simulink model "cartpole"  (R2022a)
settings: Solver=FixedStepAuto  StartTime=0.0  StopTime=20  FixedStep=Tsim  RelTol=1e-3
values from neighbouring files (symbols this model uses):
  A = [0,1,0,0 ; 0,-d1, -g*m/M,0 ; 0,0,0,1 ; 0,d1/L,q_,-d2]    [cartpole_main.m]    (also in cp_kalman.m; time_varying_LQR.m = [0,1,0,0 ; 0,-d1,f_23, f_24; 0,0,0,1; 0, f_42, f_43, f_44 ]; cp_kalman_extended.m = [0,1,0,0 ; 0,-d1,f_23, f_24; 0,0,0,1; 0, f_42, f_43, f_44 ])
  B = [0, 1.0/M, 0., -1/(M*L)].'    [cartpole_main.m]    (also in cp_kalman.m; time_varying_LQR.m = [0; cp_kalman_extended.m = [0)
  C = [1,0,0,0;0,0,1,0]    [cartpole_main.m]
  P_k_init = .01    (= 0.01)    [cartpole_main.m]
  q1 = 5e-4    (= 0.0005)    [cartpole_main.m]    (also in loop_loader.m = const(3); rob_fc.m = const(3); loop_loader_ex.m = const(3))
  q2 = 1e-3    (= 0.001)    [cartpole_main.m]    (also in loop_loader.m = const(4); rob_fc.m = const(4); loop_loader_ex.m = const(4))
  Q_ctrl = diag([10,5,20,10])    [cartpole_main.m]
  r1 = 3e-4    (= 0.0003)    [cartpole_main.m]    (also in loop_loader.m = const(1); rob_fc.m = xx; loop_loader_ex.m = const(1))
  r2 = 2e-4    (= 0.0002)    [cartpole_main.m]    (also in loop_loader.m = const(2); rob_fc.m = const(2); loop_loader_ex.m = const(2))
  R_ctrl = 10    [cartpole_main.m]
  Ts = 0.01    [cartpole_main.m]    (also in loop_loader.m; cp_kalman.m = in(4); rob_fc.m; time_varying_LQR.m = in(11))
  x0 = [0,0,0.5, 0.1]    [cartpole_main.m]
undefined symbols (not defined in the file or in its folder): K_lqr
libraries: simulink x3

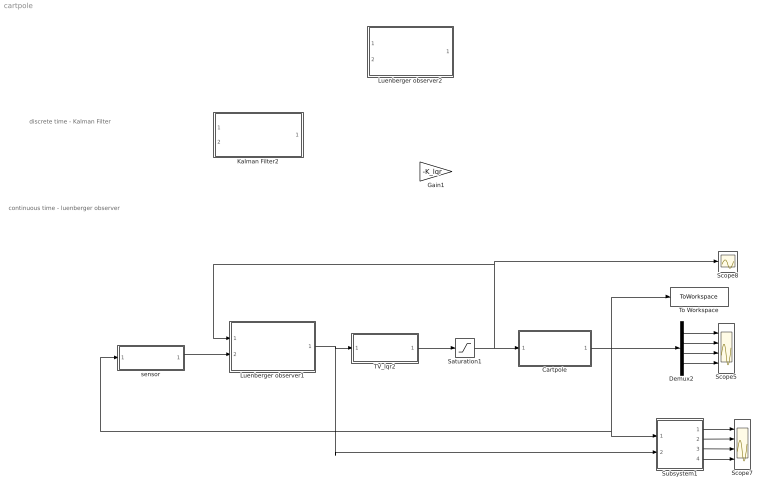
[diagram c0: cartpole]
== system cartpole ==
  note: continuous time - luenberger observer
  note: discrete time - Kalman Filter
  Cartpole : Subsystem
  Demux2 : Demux
  Gain1 : Gain  Commented=on  Gain=-K_lqr  Multiplication=Matrix(K*u)
  Kalman Filter2 : Subsystem  Commented=on  TreatAsAtomicUnit=on  SystemSampleTime=Ts
  Luenberger observer1 : Subsystem
  Luenberger observer2 : Subsystem  Commented=on
  Saturation1 : Saturate  UpperLimit=10  LowerLimit=-10
  Scope5 : Scope  NumInputPorts=4
  Scope7 : Scope  NumInputPorts=4
  Scope8 : Scope
  Subsystem1 : Subsystem
  TV_lqr2 : Subsystem  TreatAsAtomicUnit=on  SystemSampleTime=Ts
  To Workspace : ToWorkspace  VariableName=simout  SaveFormat=Timeseries  SampleTime=-1
  sensor : Subsystem
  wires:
  Subsystem1/1(x1) -> Scope7/1
  Subsystem1/3(x3) -> Scope7/3
  Subsystem1/4(x4) -> Scope7/4
  Subsystem1/2(x2) -> Scope7/2
  Demux2/4 -> Scope5/4
  Demux2/3 -> Scope5/3
  Demux2/2 -> Scope5/2
  Demux2/1 -> Scope5/1
  Saturation1/1 -> Scope8/1, Luenberger observer1/1(u), Cartpole/1(u)
  Luenberger observer1/1(x_hat) -> Subsystem1/2(x_hat), TV_lqr2/1(x)
  TV_lqr2/1(u) -> Saturation1/1
  Cartpole/1(x) -> Demux2/1, To Workspace/1, sensor/1(x), Subsystem1/1(x)
  sensor/1(y) -> Luenberger observer1/2(y)

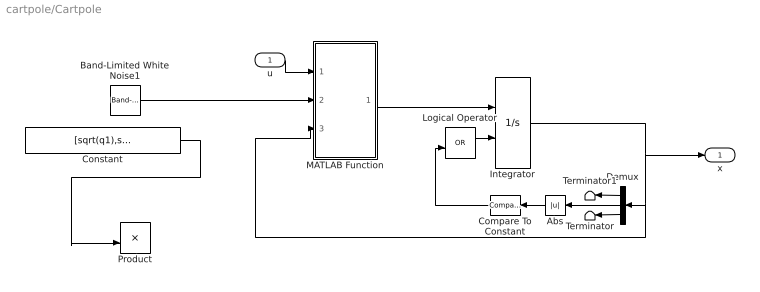
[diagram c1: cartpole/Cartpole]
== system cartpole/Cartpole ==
  u : Inport
  Abs : Abs  Commented=on
  Band-Limited White Noise1 : simulink/Sources/Band-Limited White Noise  Cov=[r1,r2]  Ts=Ts  seed=[23341]
  Compare To Constant : simulink/Logic and Bit Operations/Compare To Constant  Commented=on  relop=>=  const=1  OutDataTypeStr=boolean
  Constant : Constant  Commented=on  Value=[sqrt(q1),sqrt(q2)]
  Demux : Demux  Commented=on  Outputs=[2,1,1]
  Integrator : Integrator  ExternalReset=rising  InitialCondition=x0
  Logical Operator : Logic  Commented=on  Operator=OR  AllPortsSameDT=off  OutDataTypeStr=boolean
  MATLAB Function : MATLAB Function  TreatAsAtomicUnit=on
  Product : Product  Commented=on
  Terminator : Terminator
  Terminator1 : Terminator
  x : Outport
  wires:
  MATLAB Function/1(y) -> Integrator/1
  Integrator/1 -> x/1, MATLAB Function/3(s), Demux/1
  u/1 -> MATLAB Function/1(u)
  Compare To Constant/1 -> Logical Operator/2
  Demux/3 -> Terminator/1
  Demux/1 -> Terminator1/1
  Demux/2 -> Abs/1
  Abs/1 -> Compare To Constant/1
  Logical Operator/1 -> Integrator/2
  Constant/1 -> Product/2
  Band-Limited White Noise1/1 -> MATLAB Function/2(n)

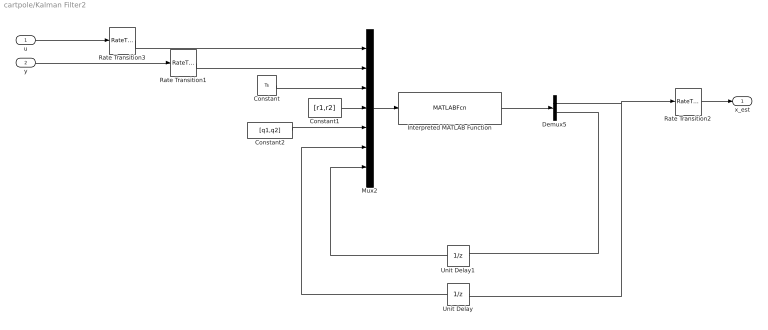
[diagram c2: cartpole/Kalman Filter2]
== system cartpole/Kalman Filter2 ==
  u : Inport
  y : Inport  Port=2
  Constant : Constant  Value=Ts
  Constant1 : Constant  Value=[r1,r2]
  Constant2 : Constant  Value=[q1,q2]
  Demux5 : Demux  Outputs=[4, 16]
  Interpreted MATLAB Function : MATLABFcn  MATLABFcn=cp_kalman  OutputDimensions=20
  Mux2 : Mux  Inputs=7
  Rate Transition1 : RateTransition  OutPortSampleTime=Ts
  Rate Transition2 : RateTransition
  Rate Transition3 : RateTransition  OutPortSampleTime=Ts
  Unit Delay : UnitDelay  InitialCondition=x0  SampleTime=-1  HasFrameUpgradeWarning=on
  Unit Delay1 : UnitDelay  InitialCondition=reshape( P_k_init*eye(4),[16,1])  SampleTime=-1  HasFrameUpgradeWarning=on
  x_est : Outport
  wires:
  Unit Delay1/1 -> Mux2/7
  Demux5/1 -> Rate Transition2/1, Unit Delay/1
  y/1 -> Rate Transition1/1
  Demux5/2 -> Unit Delay1/1
  Interpreted MATLAB Function/1 -> Demux5/1
  u/1 -> Rate Transition3/1
  Unit Delay/1 -> Mux2/6
  Mux2/1 -> Interpreted MATLAB Function/1
  Constant/1 -> Mux2/3
  Constant1/1 -> Mux2/4
  Constant2/1 -> Mux2/5
  Rate Transition3/1 -> Mux2/1
  Rate Transition1/1 -> Mux2/2
  Rate Transition2/1 -> x_est/1

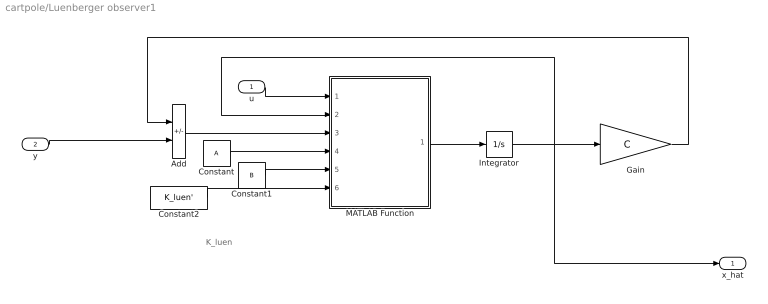
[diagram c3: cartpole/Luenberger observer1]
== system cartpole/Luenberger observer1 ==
  note: K_luen
  u : Inport
  y : Inport  Port=2
  Add : Sum  Inputs=-+
  Constant : Constant  Value=A
  Constant1 : Constant  Value=B
  Constant2 : Constant  Value=K_luen'
  Gain : Gain  Gain=C  Multiplication=Matrix(K*u)
  Integrator : Integrator  InitialCondition=[0,0,0,0]
  MATLAB Function : MATLAB Function  TreatAsAtomicUnit=on
  x_hat : Outport
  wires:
  y/1 -> Add/2
  u/1 -> MATLAB Function/1(u)
  Add/1 -> MATLAB Function/3(e)
  Gain/1 -> Add/1
  Integrator/1 -> x_hat/1, Gain/1, MATLAB Function/2(x)
  MATLAB Function/1(x_dot) -> Integrator/1
  Constant2/1 -> MATLAB Function/6(L)
  Constant1/1 -> MATLAB Function/5(B)
  Constant/1 -> MATLAB Function/4(A)

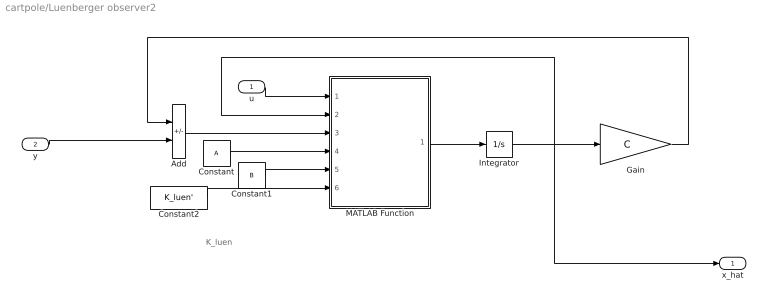
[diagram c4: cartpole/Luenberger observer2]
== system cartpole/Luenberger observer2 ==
  note: K_luen
  u : Inport
  y : Inport  Port=2
  Add : Sum  Inputs=-+
  Constant : Constant  Value=A
  Constant1 : Constant  Value=B
  Constant2 : Constant  Value=K_luen'
  Gain : Gain  Gain=C  Multiplication=Matrix(K*u)
  Integrator : Integrator  InitialCondition=[0,0,0,0]
  MATLAB Function : MATLAB Function  TreatAsAtomicUnit=on
  x_hat : Outport
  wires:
  y/1 -> Add/2
  u/1 -> MATLAB Function/1(u)
  Add/1 -> MATLAB Function/3(e)
  Gain/1 -> Add/1
  Integrator/1 -> x_hat/1, Gain/1, MATLAB Function/2(x)
  MATLAB Function/1(x_dot) -> Integrator/1
  Constant2/1 -> MATLAB Function/6(L)
  Constant1/1 -> MATLAB Function/5(B)
  Constant/1 -> MATLAB Function/4(A)

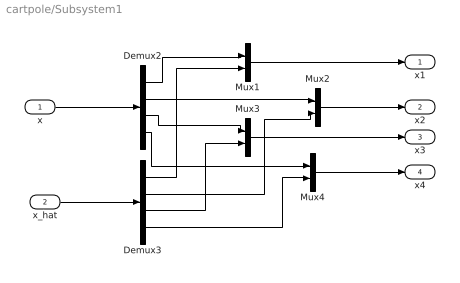
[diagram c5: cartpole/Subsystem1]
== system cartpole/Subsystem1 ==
  x : Inport
  x_hat : Inport  Port=2
  Demux2 : Demux
  Demux3 : Demux
  Mux{1..4} (4 alike) : Mux  Inputs=2
  x1 : Outport
  x2 : Outport  Port=2
  x3 : Outport  Port=3
  x4 : Outport  Port=4
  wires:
  Demux2/3 -> Mux3/1
  Demux3/4 -> Mux4/2
  x/1 -> Demux2/1
  Mux2/1 -> x2/1
  Demux2/1 -> Mux1/1
  x_hat/1 -> Demux3/1
  Demux3/2 -> Mux2/2
  Demux2/4 -> Mux4/1
  Demux3/3 -> Mux3/2
  Demux2/2 -> Mux2/1
  Mux3/1 -> x3/1
  Demux3/1 -> Mux1/2
  Mux4/1 -> x4/1
  Mux1/1 -> x1/1

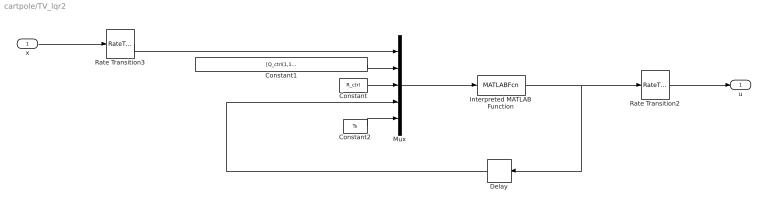
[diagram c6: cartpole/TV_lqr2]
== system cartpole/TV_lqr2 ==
  x : Inport
  Constant : Constant  Value=R_ctrl
  Constant1 : Constant  Value=[Q_ctrl(1,1),Q_ctrl(2,2),Q_ctrl(3,3),Q_ctrl(4,4)]
  Constant2 : Constant  Value=Ts
  Delay : Delay  DelayLength=1  InitialCondition=0
  Interpreted MATLAB Function : MATLABFcn  MATLABFcn=time_varying_LQR
  Mux : Mux  Inputs=5
  Rate Transition2 : RateTransition
  Rate Transition3 : RateTransition  OutPortSampleTime=Ts
  u : Outport
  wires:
  Constant2/1 -> Mux/5
  Rate Transition2/1 -> u/1
  Rate Transition3/1 -> Mux/1
  Delay/1 -> Mux/4
  Constant1/1 -> Mux/2
  Constant/1 -> Mux/3
  Mux/1 -> Interpreted MATLAB Function/1
  x/1 -> Rate Transition3/1
  Interpreted MATLAB Function/1 -> Rate Transition2/1, Delay/1

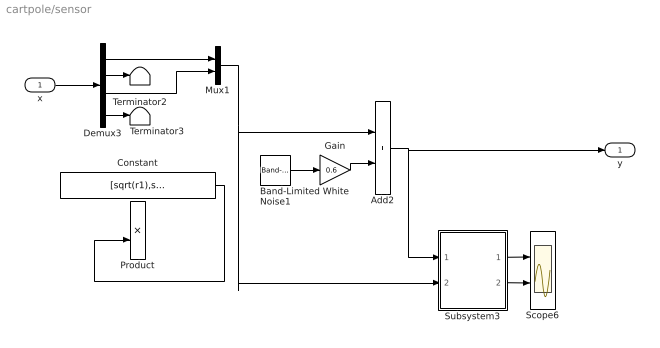
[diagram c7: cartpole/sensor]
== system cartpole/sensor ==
  x : Inport
  Add2 : Sum
  Band-Limited White Noise1 : simulink/Sources/Band-Limited White Noise  Cov=[r1,r2]  Ts=Ts  seed=[8451]
  Constant : Constant  Commented=on  Value=[sqrt(r1),sqrt(r2)]
  Demux3 : Demux
  Gain : Gain  Gain=0.6
  Mux1 : Mux  Inputs=2
  Product : Product  Commented=on
  Scope6 : Scope  NumInputPorts=2
  Subsystem3 : Subsystem
  Terminator2 : Terminator
  Terminator3 : Terminator
  y : Outport
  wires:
  Demux3/4 -> Terminator3/1
  Demux3/2 -> Terminator2/1
  Demux3/3 -> Mux1/2
  Add2/1 -> y/1, Subsystem3/1(y_noise)
  Subsystem3/2(y2) -> Scope6/2
  x/1 -> Demux3/1
  Mux1/1 -> Subsystem3/2(y), Add2/1
  Subsystem3/1(y1) -> Scope6/1
  Demux3/1 -> Mux1/1
  Constant/1 -> Product/2
  Gain/1 -> Add2/2
  Band-Limited White Noise1/1 -> Gain/1

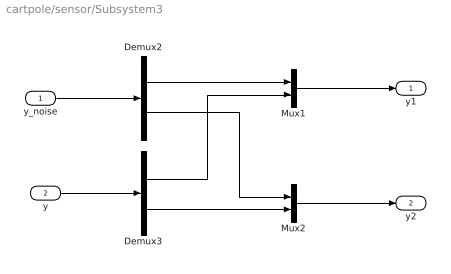
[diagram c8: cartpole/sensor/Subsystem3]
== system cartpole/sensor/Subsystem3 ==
  y_noise : Inport
  y : Inport  Port=2
  Demux2 : Demux  Outputs=2
  Demux3 : Demux  Outputs=2
  Mux1 : Mux  Inputs=2
  Mux2 : Mux  Inputs=2
  y1 : Outport
  y2 : Outport  Port=2
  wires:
  Mux1/1 -> y1/1
  Demux3/1 -> Mux1/2
  Demux2/2 -> Mux2/1
  Demux3/2 -> Mux2/2
  y/1 -> Demux3/1
  Demux2/1 -> Mux1/1
  Mux2/1 -> y2/1
  y_noise/1 -> Demux2/1

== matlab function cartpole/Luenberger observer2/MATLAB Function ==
function x_dot = fcn(u,x,e,A,B,L)

x_dot = A*x + B*u + L*e;

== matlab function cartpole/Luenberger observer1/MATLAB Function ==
function x_dot = fcn(u,x,e,A,B,L)

x_dot = A*x + B*u + L*e;

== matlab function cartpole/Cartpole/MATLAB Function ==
function y = fcn(u,n,s)

dot_x = s(2) ;
theta = s(3) ;
dot_theta = s(4) ;

m = 0.1;
L = 1;
g = 9.81;
M = 1;
d1 = 1;
d2 = 0.5;


x_ddot = u  + m*L*dot_theta^2 * sin(theta) - m*g*cos(theta) *  sin(theta) ;
x_ddot = x_ddot / ( M+m-m* cos(theta)^2 )  + n(1) - d1*dot_x;

theta_ddot = (g*sin( theta ) -  cos( theta )*x_ddot ) / L  + n(2) - d2*dot_theta ;


y = [ dot_x, x_ddot , dot_theta, theta_ddot  ];
